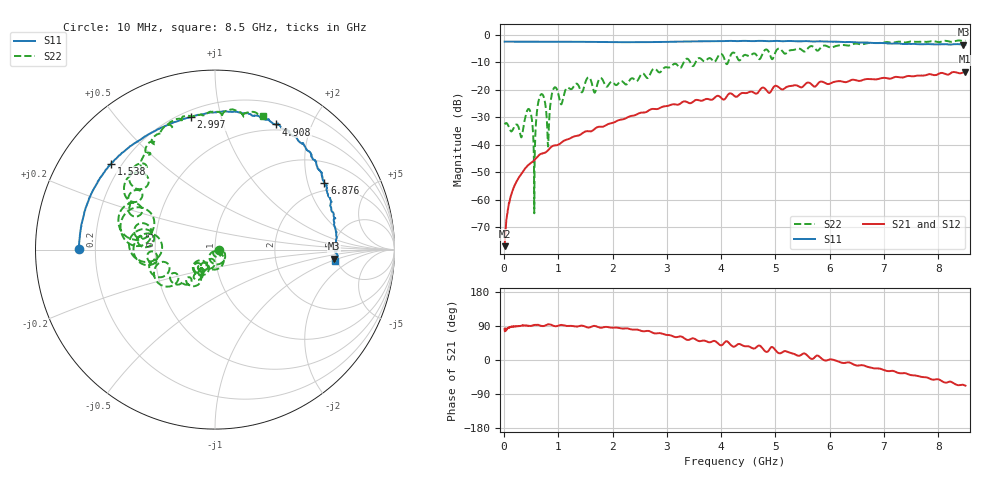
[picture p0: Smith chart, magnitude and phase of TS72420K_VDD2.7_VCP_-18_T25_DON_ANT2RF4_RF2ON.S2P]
!Agilent Technologies,E5071C,MY46417908,A.11.23
!Date: Thu Oct 03 16:41:09 2019
!Data & Calibration Information:
!Freq	S11:SOLT2(ON)	S21:SOLT2(ON)	S12:SOLT2(ON)	S22:SOLT2(ON)
!PortZ  Port1:50+j0  Port2:50+j0
!Above PortZ is port z conversion or system Z0 setting when saving the data.
!When reading, reference impedance value at option line is always used.
# Hz S dB R 50
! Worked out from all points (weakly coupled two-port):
!   1601 points, 10 MHz to 8.5 GHz, reference 50 ohm
!   highest |S21| = -13.40 dB at 8.495 GHz (marker M1); lowest = -77.0 dB at 10 MHz (marker M2)
!   lowest |S11| = -3.5 dB at 8.463 GHz (marker M3), VSWR 5.00, Z = 241 - j44.5 ohm
!   |S11| at or under -10 dB: nowhere
!   |S22| runs from -65.0 to -2.0 dB; largest |S21 - S12| = 0.0023
!   S11 on the Smith chart (normalised r, x): 10 MHz: 0.14, +0.00; 1.538 GHz: 0.16, +0.35; 2.997 GHz: 0.24, +0.81; 4.908 GHz: 0.43, +1.52; 6.876 GHz: 1.68, +2.56; 8.5 GHz: 4.82, -1.13
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1e7  -2.38 179.8  -76.98 81.7  -80.46 75.9  -32.56 0.2
1.214312e8  -2.41 176.6  -59.04 87.5  -58.87 87.4  -34.95 -23.0
3.389875e8  -2.42 170.5  -50.04 91.2  -50.06 90.6  -35.76 -5.8
4.55725e8  -2.42 167.4  -47.23 90.1  -47.24 90.2  -26.95 -61.9
5.6185e8  -2.42 164.5  -45.56 92.2  -45.51 92.4  -48.17 39.9
6.838938e8  -2.43 161.5  -43.26 90.0  -43.27 90.1  -21.57 -66.7
8.059375e8  -2.42 158.2  -42.12 94.0  -42.13 93.8  -39.39 -114.4
9.279812e8  -2.43 155.3  -40.27 89.5  -40.26 89.5  -19.13 -86.5
1.050025e9  -2.45 152.3  -39.32 92.5  -39.30 92.5  -25.27 -108.6
1.426769e9  -2.48 143.0  -36.04 90.5  -36.04 90.5  -20.81 -125.5
1.5382e9  -2.48 140.4  -35.04 86.0  -35.03 86.0  -15.60 -122.0
1.670856e9  -2.52 137.2  -34.21 90.0  -34.21 89.9  -21.01 -129.5
2.843538e9  -2.53 104.5  -26.86 70.9  -26.85 70.8  -13.46 -133.6
2.997419e9  -2.49 100.2  -25.92 66.2  -25.92 66.1  -11.73 -134.9
4.255e9  -2.17 75.2  -22.38 36.0  -22.36 35.9  -6.79 168.1
4.907669e9  -2.20 63.9  -20.82 31.7  -20.75 31.4  -7.64 150.2
5.671769e9  -2.34 52.7  -18.11 2.8  -18.03 3.1  -4.04 139.2
6.876288e9  -2.92 31.4  -16.13 -22.3  -16.12 -22.4  -2.92 114.6
7.088538e9  -3.08 26.9  -15.88 -29.5  -15.86 -29.0  -2.61 110.0
8.462856e9  -3.52 -4.4  -13.60 -65.6  -13.64 -66.0  -2.14 71.1
8.494694e9  -3.47 -5.3  -13.40 -67.4  -13.44 -67.8  -2.06 70.3
8.5e9  -3.46 -5.5  -13.40 -67.7  -13.44 -68.2  -2.05 70.2
